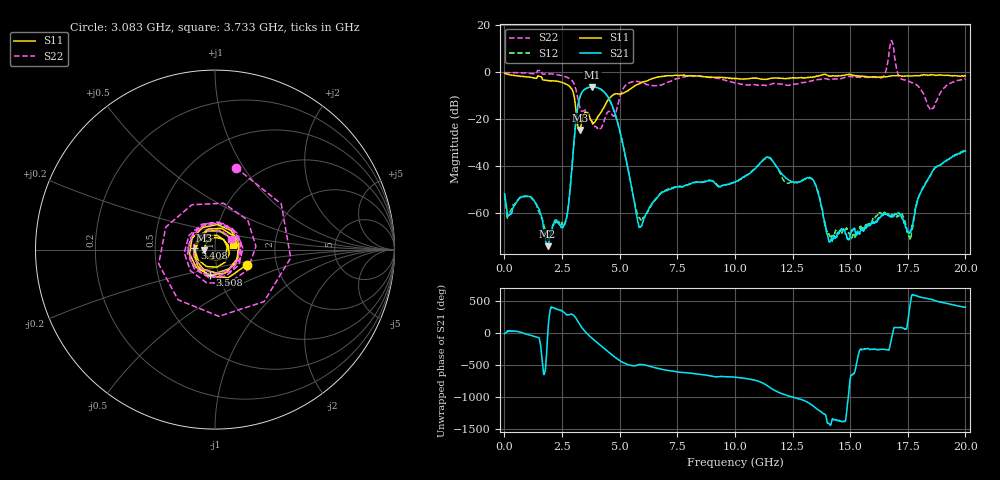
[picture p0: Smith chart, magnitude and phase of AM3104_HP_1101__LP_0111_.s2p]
!Created with skrf (http://scikit-rf.org).
# Hz S RI R 50.0
!freq ReS11 ImS11 ReS21 ImS21 ReS12 ImS12 ReS22 ImS22
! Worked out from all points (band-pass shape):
!   1601 points, 10 MHz to 20 GHz, reference 50 ohm
!   highest |S21| = -6.14 dB at 3.821 GHz (marker M1); lowest = -74.0 dB at 1.872 GHz (marker M2)
!   |S21| within 3 dB of the highest: 3.327 GHz to 4.398 GHz (1.07 GHz wide, 27.7 % of centre)
!   lowest |S11| = -24.5 dB at 3.271 GHz (marker M3), VSWR 1.13, Z = 44.4 - j0.278 ohm
!   |S11| at or under -10 dB: 3.022 GHz to 4.666 GHz (1.643 GHz wide, 42.8 % of centre)
!   |S22| runs from -23.9 to 13.6 dB; largest |S21 - S12| = 0.035
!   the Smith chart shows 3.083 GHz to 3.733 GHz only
!   S11 on the Smith chart (normalised r, x): 3.083 GHz: 1.41, -0.25; 3.408 GHz: 0.79, +0.01; 3.508 GHz: 0.91, -0.26; 3.733 GHz: 1.22, +0.06
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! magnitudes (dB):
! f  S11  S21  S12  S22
! 10 MHz  -0.4  -51.7  -52.2  -0.1
! 1.209 GHz  -2.2  -53.6  -53.8  -0.5
! 1.872 GHz  -3.5  -74.0  -70.8  -0.7
! 2.671 GHz  -4.9  -62.7  -62.7  -1.9
! 3.083 GHz  -14.1  -22.7  -22.6  -6.6
! 3.271 GHz  -24.5  -10.6  -10.7  -14.9
! 3.346 GHz  -21.6  -8.8  -8.9  -16.5
! 3.408 GHz  -18.8  -7.9  -7.9  -16.4
! 3.508 GHz  -16.8  -7.0  -7.1  -15.9
! 3.733 GHz  -20.0  -6.2  -6.2  -19.6
! 3.821 GHz  -21.5  -6.1  -6.2  -21.6
! 4.758 GHz  -9.3  -16.3  -16.4  -18.6
! 5.857 GHz  -4.8  -66.0  -61.7  -4.0
! 6.682 GHz  -1.9  -52.7  -52.3  -5.6
! 10.01 GHz  -2.7  -46.8  -46.7  -4.5
! 11.43 GHz  -2.8  -35.9  -36.2  -5.5
! 13.34 GHz  -2.1  -45.3  -45.3  -3.6
! 14.14 GHz  -1.6  -71.8  -70.6  -3.0
! 16.68 GHz  -1.6  -60.8  -60.9  7.1
! 17.6 GHz  -1.5  -68.0  -71.3  -4.0
! 18.5 GHz  -1.1  -43.6  -43.6  -16.1
! 20 GHz  -1.4  -33.5  -32.9  -2.7
